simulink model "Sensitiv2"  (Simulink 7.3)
settings: Solver=ode45  StartTime=0.0  StopTime=10.0  RelTol=1e-3
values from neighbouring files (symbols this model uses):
  Kl3 = INFO.KFI(:,1:7)    [run.m]
undefined symbols (not defined in the file or in its folder): An, Bn, Cn, Dn

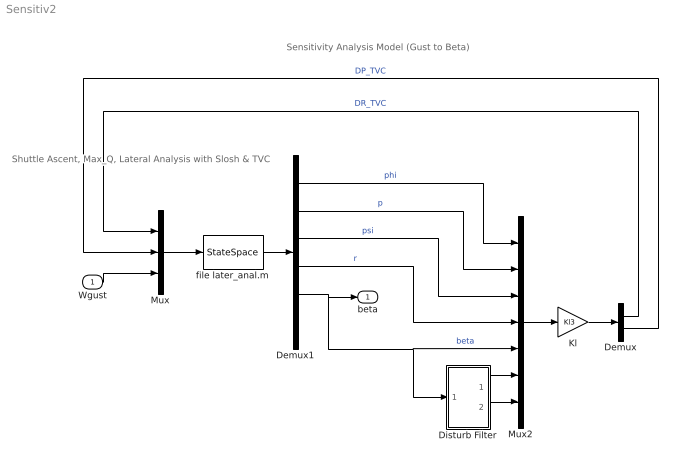
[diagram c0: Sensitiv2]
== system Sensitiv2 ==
  note: Shuttle Ascent, Max_Q, Lateral Analysis with Slosh & TVC
  note: Sensitivity Analysis Model (Gust to Beta)
  Wgust : Inport  OutDataType=sfix(16)  OutScaling=2^0
  Demux : Demux  Outputs=2
  Demux1 : Demux  Outputs=6
  Disturb Filter : Subsystem
  Kl : Gain  Gain=Kl3  Multiplication=Matrix(K*u)  ParameterDataType=sfix(16)  ParameterScaling=2^0  OutDataType=sfix(16)  OutScaling=2^0
  Mux : Mux  Inputs=3
  Mux2 : Mux  Inputs=7
  file later_anal.m : StateSpace  A=An  B=Bn  C=Cn  D=Dn
  beta : Outport  OutDataType=sfix(16)  OutScaling=2^0
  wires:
  Mux/1 -> file later_anal.m/1
  Kl/1 -> Demux/1
  Demux/1 -> Mux/1  "DR_TVC"
  file later_anal.m/1 -> Demux1/1
  Mux2/1 -> Kl/1
  Disturb Filter/1(x1) -> Mux2/6
  Disturb Filter/2(x2) -> Mux2/7
  Demux1/1 -> Mux2/1  "phi"
  Demux1/2 -> Mux2/2  "p"
  Demux1/3 -> Mux2/3  "psi"
  Demux1/4 -> Mux2/4  "r"
  Demux/2 -> Mux/2  "DP_TVC"
  Wgust/1 -> Mux/3
  Demux1/5 -> beta/1, Mux2/5, Disturb Filter/1(bet)  "beta"

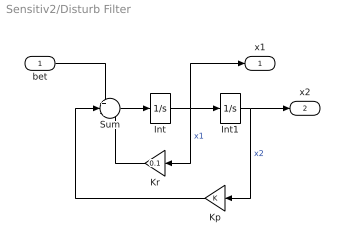
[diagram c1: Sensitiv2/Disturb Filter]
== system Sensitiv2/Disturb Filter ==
  bet : Inport  OutDataType=sfix(16)  OutScaling=2^0
  Int : Integrator
  Int1 : Integrator
  Kp : Gain  ParameterDataType=sfix(16)  ParameterScaling=2^0  OutDataType=sfix(16)  OutScaling=2^0
  Kr : Gain  Gain=0.1  ParameterDataType=sfix(16)  ParameterScaling=2^0  OutDataType=sfix(16)  OutScaling=2^0
  Sum : Sum  Inputs=+--  OutDataType=sfix(16)  OutScaling=2^0
  x1 : Outport  OutDataType=sfix(16)  OutScaling=2^0
  x2 : Outport  Port=2  OutDataType=sfix(16)  OutScaling=2^0
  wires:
  Int/1 -> Int1/1, Kr/1, x1/1  "x1"
  Sum/1 -> Int/1
  Int1/1 -> Kp/1, x2/1  "x2"
  Kr/1 -> Sum/3
  Kp/1 -> Sum/2
  bet/1 -> Sum/1
